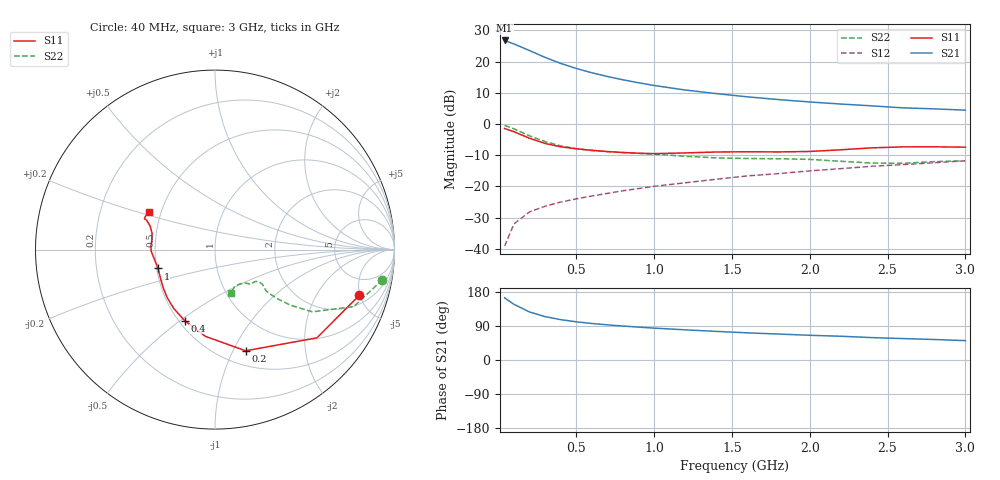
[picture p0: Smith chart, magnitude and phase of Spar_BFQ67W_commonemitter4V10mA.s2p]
! Filename:  BFQ67WC.S2P  Version:  4.0
! NXP part #: BFQ67W  Date: Jun 1994
! Bias condition: Vce=4V, Ic=10mA
#  MHz  S  MA  R  50
! Freq  S11  S21  S12  S22  !GUM [dB]
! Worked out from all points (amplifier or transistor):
!   21 points, 40 MHz to 3 GHz, reference 50 ohm
!   highest |S21| = 26.7 dB at 40 MHz (marker M1)
!   |S21| within 3 dB of that: start of sweep to 188.5 MHz
!   unconditionally stable (mu >= 1): 813 MHz to end of sweep
!   at 300 MHz: K = 0.64, MSG = 23.8 dB, |S12| = -26.4 dB
!   at 1 GHz: K = 1.06, MAG = 14.7 dB, |S12| = -20.0 dB
!   at 3 GHz: K = 1.03, MAG = 7.0 dB, |S12| = -11.8 dB
!   lowest NFmin = 1.70 dB at 1 GHz
!   S11 on the Smith chart (normalised r, x): 40 MHz: 2.81, -4.95; 200 MHz: 0.65, -1.12; 400 MHz: 0.53, -0.52; 1 GHz: 0.51, -0.12; 3 GHz: 0.43, +0.22
40  0.844 -17.5  21.74 164.0  0.011 79.8  0.948 -10.2
100  0.751 -40.9  19.11 146.9  0.025 68.1  0.836 -22.3
200  0.589 -73.2  14.96 126.8  0.039 58.9  0.644 -32.6
300  0.486 -96.4  11.64 114.5  0.048 56.6  0.521 -36.4
400  0.43 -113.2  9.326 106.5  0.056 57.2  0.446 -38.1
500  0.4 -125.2  7.742 100.8  0.063 58.4  0.401 -38.8
600  0.378 -134.6  6.607 96.4  0.07 60.2  0.375 -38.9
700  0.361 -142.3  5.754 92.8  0.077 62.0  0.359 -38.6
800  0.348 -149.0  5.091 89.6  0.085 63.6  0.348 -37.8
900  0.339 -155.6  4.566 86.8  0.092 64.7  0.338 -37.0
1000  0.334 -161.7  4.131 84.1  0.1 65.7  0.328 -36.3
1200  0.343 -171.8  3.495 79.6  0.114 67.4  0.303 -36.1
1400  0.355 -178.2  3.06 75.5  0.13 68.8  0.286 -38.4
1600  0.358 177.3  2.716 71.6  0.147 69.1  0.279 -42.3
1800  0.356 172.0  2.453 68.5  0.16 70.0  0.277 -44.2
2000  0.362 165.4  2.247 65.2  0.177 70.5  0.27 -45.2
2200  0.385 160.0  2.082 62.7  0.192 71.2  0.252 -47.5
2400  0.414 156.8  1.947 59.1  0.21 71.2  0.236 -53.9
2600  0.429 156.4  1.807 56.5  0.223 70.7  0.234 -62.4
2800  0.43 154.9  1.743 54.1  0.239 71.2  0.249 -67.4
3000  0.424 150.4  1.661 51.1  0.257 70.9  0.256 -69.7
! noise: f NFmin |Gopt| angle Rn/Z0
1000  1.7  0.23  86.5  0.26
